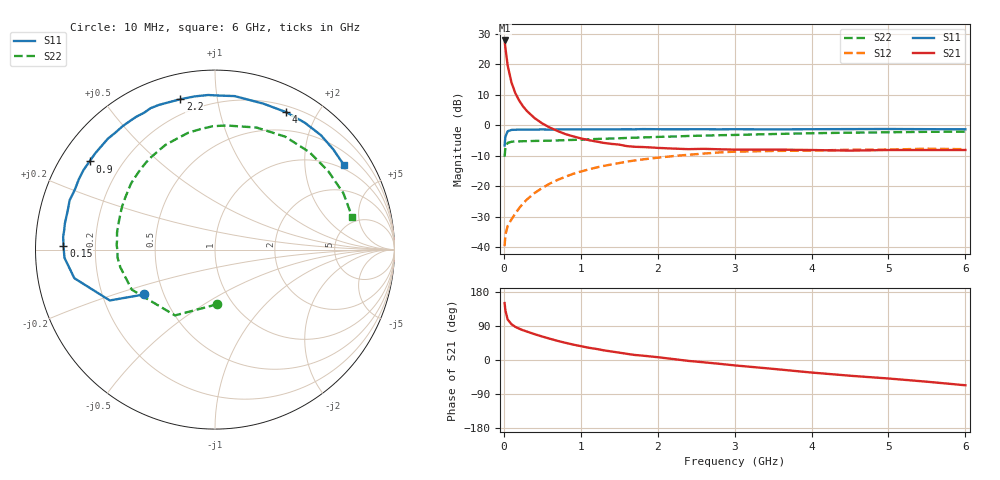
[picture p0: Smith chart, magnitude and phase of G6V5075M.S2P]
! SIEMENS Small Signal Semiconductors
! BFG193
! Si NPN RF Bipolar Junction Transistor in SOT223
! VCE = 0.5 V  IC = 75 mA
! Common Emitter S-Parameters:  August  1996
# GHz  S  MA  R  50
!  f  S11  S21  S12  S22
! GHz  MAG  ANG  MAG  ANG  MAG  ANG  MAG  ANG
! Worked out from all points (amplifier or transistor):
!   36 points, 10 MHz to 6 GHz, reference 50 ohm
!   highest |S21| = 27.8 dB at 10 MHz (marker M1)
!   |S21| within 3 dB of that: start of sweep to 23.1 MHz
!   unconditionally stable (mu >= 1): start of sweep to 18.85 MHz; 79.62 MHz to end of sweep
!   at 250 MHz: K = 1.38, MAG = 12.3 dB, |S12| = -25.6 dB
!   at 1.4 GHz: K = 1.28, MAG = 0.2 dB, |S12| = -12.9 dB
!   at 6 GHz: K = 1.07, MAG = -1.7 dB, |S12| = -7.8 dB
!   S11 on the Smith chart (normalised r, x): 10 MHz: 0.39, -0.25; 150 MHz: 0.08, +0.01; 900 MHz: 0.09, +0.31; 2.2 GHz: 0.12, +0.79; 4 GHz: 0.27, +1.61; 6 GHz: 0.87, +3.12
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0.01  0.4677 -147.7  24.64 150.2  0.0104 56.7  0.305 -87.7
0.02  0.6511 -154.2  18.7 131.0  0.016 44.2  0.4292 -121.3
0.05  0.7996 -168.5  9.525 106.7  0.0223 40.4  0.5146 -154.3
0.1  0.8401 -176.9  4.988 94.3  0.0288 47.9  0.5366 -169.4
0.15  0.8444 178.5  3.351 87.3  0.0357 53.3  0.5451 -175.6
0.2  0.8489 175.2  2.54 82.6  0.0439 57.2  0.5436 -179.4
0.25  0.8472 172.7  2.038 78.5  0.0522 59.5  0.5486 177.2
0.3  0.849 170.1  1.714 75.0  0.0606 60.8  0.548 174.9
0.4  0.8487 165.3  1.311 68.1  0.0776 61.7  0.554 170.1
0.5  0.8553 161.2  1.071 61.9  0.0939 60.3  0.5561 166.0
0.6  0.8494 157.0  0.914 56.0  0.111 58.8  0.5594 162.3
0.7  0.854 152.5  0.804 50.4  0.1272 57.0  0.5645 158.7
0.9  0.8545 144.9  0.659 40.7  0.1596 51.9  0.5759 151.3
1.1  0.856 137.6  0.572 32.4  0.1883 47.1  0.5885 144.7
1.6  0.8605 120.7  0.455 16.3  0.2534 32.9  0.6199 128.0
2.2  0.8598 103.0  0.415 2.6  0.3124 16.1  0.6536 108.9
2.8  0.8586 87.2  0.404 -10.0  0.3585 0.2  0.6875 91.0
3.5  0.8566 71.7  0.4 -23.4  0.3791 -18.3  0.7184 71.2
4  0.8622 62.7  0.393 -33.1  0.3846 -27.5  0.7409 58.1
4.5  0.8662 54.6  0.384 -41.5  0.3974 -36.6  0.7563 45.8
5.5  0.8636 40.3  0.393 -57.3  0.4127 -57.1  0.7813 23.7
6  0.8592 33.3  0.393 -66.7  0.4055 -68.7  0.7851 13.5
